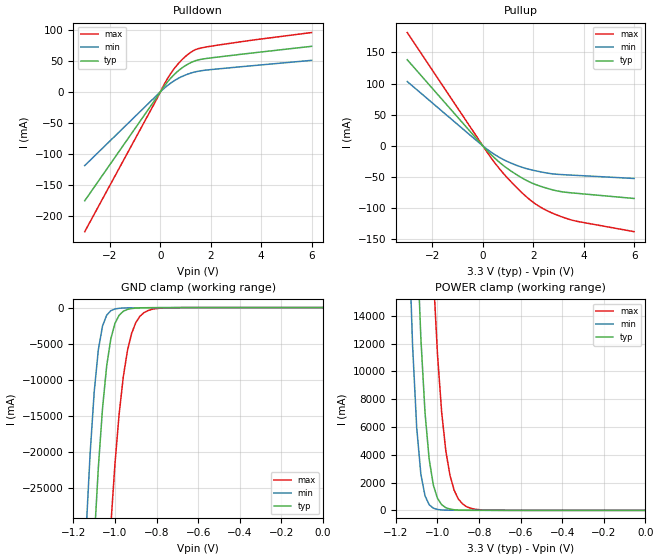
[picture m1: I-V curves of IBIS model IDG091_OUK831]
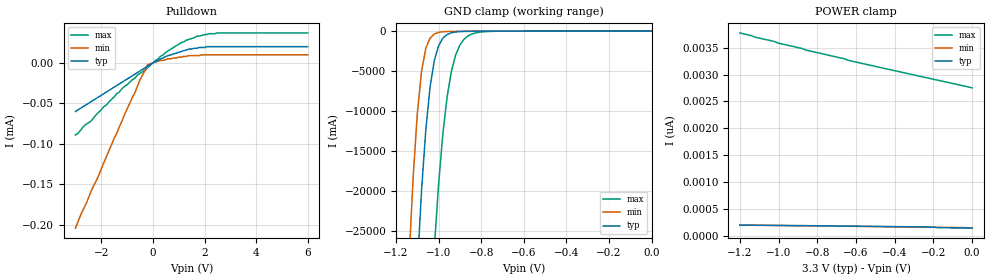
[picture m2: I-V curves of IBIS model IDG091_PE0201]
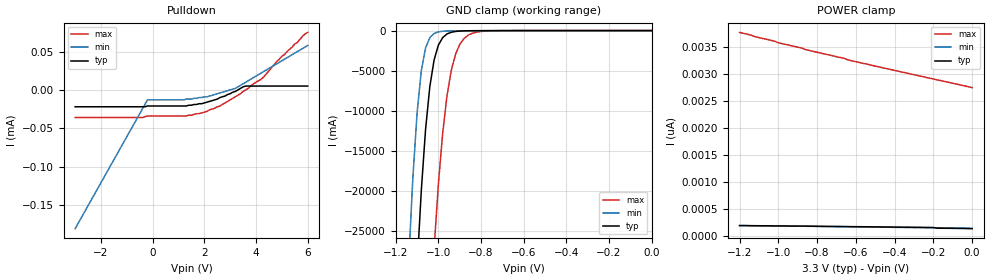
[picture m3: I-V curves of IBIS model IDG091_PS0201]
[IBIS Ver]   2.1
[File name]   dac5674.ibs
[File Rev]   1.0
[Date]   08 DEC 2004
[Source]   Preliminary Model
[Notes]
   Technology type GS30
[Disclaimer]   Please be aware that in the absence of a written agreement
|   Texas Instruments(TI) assumes no liability for:
|   (1) The accuracy of the IBIS models provided to your company
|   (2) The proper functioning of these Models in your design
|   or for any resulting applications;or
|   property rights resulting from your use of these models.
|   TI provides IBIS Models as a service to our customers and
|   therefore reserves the right to limit distribution of the
|   Models.
[Copyright]   Property of Texas Instruments Incorporated.
|   Unauthorised reproduction and/or distribution is strictly.
|   prohibited.
|   This product is protected under copyright law and trade
|   secret law as an unpublished work.
|   Created 1999,(C) Copyright 1999-2001,
|   Texas Instruments Incorporated., All Rights Reserved.
|   These commodities are under the U.S.
|   Government distribution license control.As such,they are not
|   to be re-exported without the prior approval of the U.S.
|   Department of Commerce.
[Component]   dac5674
[Manufacturer]   Texas Instruments
[Package]
|   typ   min   max
R_pkg   0.114   0.028   0.162
L_pkg   3.172nH   2.482nH   4.042nH
C_pkg   0.140pF   0.089pF   0.217pF
[Pin]   signal_name   model_name   R_pin   L_pin   C_pin
   1   DGND   GND   0.083   3.524nH   0.213pF
   2   DGND   GND   0.153   3.828nH   0.113pF
   3   D13   IDG091_PE0201   0.147   3.682nH   0.108pF
   4   D12   IDG091_PE0201   0.143   3.569nH   0.104pF
   5   D11   IDG091_PE0201   0.140   3.487nH   0.103pF
   6   D10   IDG091_PE0201   0.073   3.022nH   0.199pF
   7   D9   IDG091_PE0201   0.139   3.401nH   0.104pF
   8   D8   IDG091_PE0201   0.140   2.975nH   0.197pF
   9   D7   IDG091_PE0201   0.140   3.391nH   0.098pF
   10   D6   IDG091_PE0201   0.140   3.410nH   0.103pF
   11   D5   IDG091_PE0201   0.141   3.461nH   0.105pF
   12   D4   IDG091_PE0201   0.073   3.102nH   0.206pF
   13   D3   IDG091_PE0201   0.073   3.174nH   0.211pF
   14   D2   IDG091_PE0201   0.073   3.260nH   0.218pF
   15   D1   IDG091_PE0201   0.078   3.360nH   0.223pF
   16   D0   IDG091_PE0201   0.028   2.456nH   0.090pF
   17   HP1   IDG091_PE0201   0.153   3.934nH   0.103pF
   18   HP2   IDG091_PE0201   0.076   3.327nH   0.217pF
   19   DGND   GND   0.076   3.233nH   0.212pF
   20   IOGND   GND   0.073   3.154nH   0.206pF
   21   DVDD   POWER   0.073   3.096nH   0.204pF
   22   IODVDD   POWER   0.073   3.051nH   0.202pF
   23   X4   IDG091_PE0201   0.073   3.018nH   0.201pF
   24   DGND   GND   0.143   3.416nH   0.105pF
   25   PLLLOCK   OUK831   0.073   2.993nH   0.198pF
   26   RESET   IDG091_PE0201   0.073   3.008nH   0.199pF
   27   DIV1   IDG091_PE0201   0.141   3.462nH   0.105pF
   28   DIV0   IDG091_PE0201   0.143   3.533nH   0.107pF
   29   CLK   IOH121   0.075   3.190nH   0.210pF
   30   CLKC   IOH121   0.075   3.272nH   0.215pF
   31   CLKGND   GND   0.153   3.839nH   0.112pF
   32   CLKVDD   POWER   0.028   2.477nH   0.094pF
   33   PLLGND   GND   0.153   2.919nH   0.089pF
   34   PLLVDD   POWER   0.145   2.784nH   0.095pF
   35   LPF   IOH121   0.140   2.700nH   0.089pF
   36   SLEEP   IDG091_PE0201   0.072   2.292nH   0.163pF
   37   AGND   GND   0.072   2.270nH   0.164pF
   38   EXTLO   IOH121   0.072   2.255nH   0.163pF
   39   EXTIO   IOH121   0.072   2.252nH   0.161pF
   40   BIASJ   IOH121   0.140   2.675nH   0.091pF
   41   AGND   GND   0.140   2.662nH   0.093pF
   42   IOUT2   IOH121   0.072   2.242nH   0.160pF
   43   IOUT1   IOH121   0.138   2.652nH   0.090pF
   44   AGND   GND   0.139   2.671nH   0.090pF
   45   AVDD   POWER   0.142   2.710nH   0.091pF
   46   AVDD   POWER   0.145   2.768nH   0.093pF
   47   DVDD   POWER   0.150   2.854nH   0.097pF
   48   DVDD   POWER   0.077   2.482nH   0.163pF
| Models and submodels in the file (5): IDG091_OUK831 (I/O), IDG091_PE0201 (Input), IDG091_PS0201 (Input), OUK831 (3-state), IOH121 (Input)
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[Model]   IDG091_OUK831
Model_type   I/O
Enable   Active-Low
Polarity   Non-Inverting
| signals   A, GZ, Y
Vinl = 0.8V
Vinh = 2.0V
Vmeas = 1.5
|   typ   min   max
C_comp   3.5921p   3.4389p   4.1227p
|   typ   min   max
[Temperature Range]   25   -40.0   125
|   typ   min   max
[Voltage Range]   3.30V   3.00V   3.60V
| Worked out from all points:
|   slope of the pulldown table from 0 to 0.495 V, typ, clamps not added: 19.3 ohm
|   slope of the pullup table from 0 to 0.495 V, typ, clamps not added: 24.2 ohm
|   GND clamp passes 1 mA (typ) near -0.58 V on its own axis
|   POWER clamp passes 1 mA (typ) near -0.64 V on its own axis
[Pulldown]
|   Voltage   I(typ)   I(min)   I(max)
-3V       -175.9mA   -119.1mA   -225.8mA
-200mV    -12.18mA   -7.956mA   -16.01mA
200mV     11.61mA    7.405mA    15.55mA
400mV     21.52mA    13.77mA    28.85mA
600mV     29.89mA    19.16mA    40.1mA
1V        42.47mA    27.25mA    57.28mA
1.3V      48.84mA    31.34mA    66.22mA
1.7V      53.08mA    34.51mA    71.52mA
3.6V      62.5mA     41.98mA    83.19mA
6V        73.47mA    50.83mA    95.74mA
[GND_clamp]
|   Voltage   I(typ)   I(min)   I(max)
-1.2V     -102.7A    -74.41A    -154.1A
-1.14V    -57.55A    -31.62A    -106.7A
-1.1V     -32.35A    -11.69A    -77.65A
-1.08V    -22.13A    -5.816A    -64.19A
-1.06V    -13.97A    -2.559A    -51.65A
-1.04V    -8.085A    -1.052A    -40.23A
-1.02V    -4.316A    -431.8mA   -30.14A
-980mV    -1.059A    -97.69mA   -14.73A
-960mV    -513.4mA   -60.94mA   -9.568A
-920mV    -131.1mA   -37.25mA   -3.566A
-880mV    -45.19mA   -28.49mA   -1.203A
0V        -130.5pA   -109.2pA   -2.072nA
[Pullup]
|   Voltage   I(typ)   I(min)   I(max)
-3V       138.1mA    103.2mA    181.7mA
-200mV    9.146mA    6.727mA    12.21mA
300mV     -12.88mA   -9.22mA    -17.63mA
900mV     -34.12mA   -23.64mA   -48.03mA
1.7V      -54.7mA    -36.06mA   -80.58mA
2.1V      -62.01mA   -39.98mA   -93.36mA
2.4V      -66.16mA   -42.43mA   -100.8mA
2.9V      -71.73mA   -45.34mA   -110.1mA
3.3V      -74.37mA   -46.38mA   -116.1mA
3.8V      -76.3mA    -47.46mA   -121.4mA
6V        -84.26mA   -52.21mA   -137.4mA
[POWER_clamp]
|   Voltage   I(typ)   I(min)   I(max)
-1.2V     83.43A     59.64A     127.8A
-1.14V    41.42A     20.8A      82.7A
-1.12V    29.85A     11.95A     68.94A
-1.1V     20.06A     5.958A     56.04A
-1.08V    12.41A     2.607A     44.19A
-1.06V    7.027A     1.048A     33.6A
-1.04V    3.679A     406.1mA    24.47A
-1.02V    1.819A     157.9mA    16.99A
-960mV    192.4mA    15.59mA    4.285A
-920mV    44.41mA    7.991mA    1.453A
-880mV    12.4mA     6.125mA    468.3mA
0V        154.5pA    161.2pA    3.029nA
[Ramp]
|   I(typ)   I(min)   I(max)
dV/dt_r   1.267/1.474n   0.957/2.769n   1.564/0.824n
dV/dt_f   1.332/1.513n   0.961/2.653n   1.616/0.826n
[Model]   IDG091_PE0201
Model_type   Input
Polarity   Non-Inverting
| signals   A, Y
Vinl = 0.8V
Vinh = 2.0V
|   typ   min   max
C_comp   3.016p   2.9215p   3.4873p
|   typ   min   max
[Temperature Range]   25   -40.0   125
|   typ   min   max
[Voltage Range]   3.30V   3.00V   3.60V
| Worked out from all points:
|   slope of the pulldown table from 0 to 0.495 V, typ, clamps not added: 62.7 kohm
|   GND clamp passes 1 mA (typ) near -0.58 V on its own axis
[Pulldown]
|   Voltage   I(typ)   I(min)   I(max)
-3V       -60uA      -204uA     -89uA
-2.6V     -52uA      -175uA     -76uA
-2.4V     -48uA      -159uA     -72uA
-2.1V     -42uA      -139uA     -61uA
-1.1V     -22uA      -64uA      -29uA
-500mV    -10uA      -21uA      -13uA
-200mV    -4uA       -2uA       -6uA
500mV     8uA        4uA        13uA
1.1V      14uA       7uA        25uA
1.7V      18uA       9uA        33uA
2.5V      20uA       10uA       37uA
6V        20uA       10uA       37uA
[GND_clamp]
|   Voltage   I(typ)   I(min)   I(max)
-1.2V     -98.78A    -71.42A    -148.8A
-1.14V    -54.21A    -29.33A    -101.8A
-1.1V     -29.69A    -10.34A    -73.18A
-1.08V    -19.94A    -5.01A     -60A
-1.06V    -12.33A    -2.162A    -47.8A
-1.04V    -6.983A    -880.6mA   -36.79A
-1.02V    -3.664A    -361.6mA   -27.18A
-980mV    -884.2mA   -83.74mA   -12.87A
-960mV    -428mA     -53.16mA   -8.232A
-920mV    -110.2mA   -33.2mA    -3A
-880mV    -38.87mA   -25.56mA   -1.002A
0V        -427.6fA   -2.728fA   -107pA
[POWER_clamp]
|   Voltage   I(typ)   I(min)   I(max)
-1.2V     197.2pA    197.2pA    3.775nA
-1.14V    194.5pA    194.5pA    3.723nA
-1.12V    194.5pA    193.6pA    3.695nA
-1.02V    191pA      190.1pA    3.613nA
-1V       191pA      189.2pA    3.583nA
-880mV    187.4pA    184.7pA    3.485nA
-860mV    187.4pA    184.7pA    3.456nA
-660mV    178.5pA    175.9pA    3.293nA
-640mV    178.1pA    175pA      3.265nA
-200mV    160.8pA    156.8pA    2.912nA
-180mV    148.8pA    155.9pA    2.896nA
0V        139.9pA    145.7pA    2.752nA
[Model]   IDG091_PS0201
Model_type   Input
Polarity   Non-Inverting
| signals   A, Y
Vinl = 0.8V
Vinh = 2.0V
|   typ   min   max
C_comp   2.9577p   2.8282p   3.4534p
|   typ   min   max
[Temperature Range]   25   -40.0   125
|   typ   min   max
[Voltage Range]   3.30V   3.00V   3.60V
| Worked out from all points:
|   GND clamp passes 1 mA (typ) near -0.58 V on its own axis
[Pulldown]
|   Voltage   I(typ)   I(min)   I(max)
-3V       -22uA      -181uA     -36uA
-400mV    -22uA      -25uA      -36uA
-200mV    -21uA      -13uA      -34uA
1.3V      -21uA      -12uA      -34uA
1.9V      -18uA      -10uA      -30uA
2.6V      -10uA      -4uA       -21uA
3.2V      -2uA       2uA        -9uA
3.6V      5uA        10uA       0A
4.3V      5uA        24uA       17uA
5V        5uA        38uA       44uA
5.8V      5uA        54uA       70uA
6V        5uA        58uA       75uA
[GND_clamp]
|   Voltage   I(typ)   I(min)   I(max)
-1.2V     -98.78A    -71.42A    -148.8A
-1.14V    -54.21A    -29.33A    -101.8A
-1.1V     -29.69A    -10.34A    -73.18A
-1.08V    -19.94A    -5.01A     -60A
-1.06V    -12.33A    -2.162A    -47.8A
-1.04V    -6.983A    -880.6mA   -36.79A
-1.02V    -3.664A    -361.6mA   -27.18A
-980mV    -884.2mA   -83.74mA   -12.87A
-960mV    -428mA     -53.16mA   -8.232A
-920mV    -110.2mA   -33.2mA    -3A
-880mV    -38.87mA   -25.56mA   -1.002A
0V        -427.6fA   -2.728fA   -107pA
[POWER_clamp]
|   Voltage   I(typ)   I(min)   I(max)
-1.2V     197.2pA    197.2pA    3.775nA
-1.14V    194.5pA    194.5pA    3.723nA
-1.12V    194.5pA    193.6pA    3.695nA
-1.02V    191pA      190.1pA    3.613nA
-1V       191pA      189.2pA    3.583nA
-880mV    187.4pA    184.7pA    3.485nA
-860mV    187.4pA    184.7pA    3.456nA
-660mV    178.5pA    175.9pA    3.293nA
-640mV    178.1pA    175pA      3.265nA
-200mV    160.8pA    156.8pA    2.912nA
-180mV    148.8pA    155.9pA    2.896nA
0V        139.9pA    145.7pA    2.752nA
